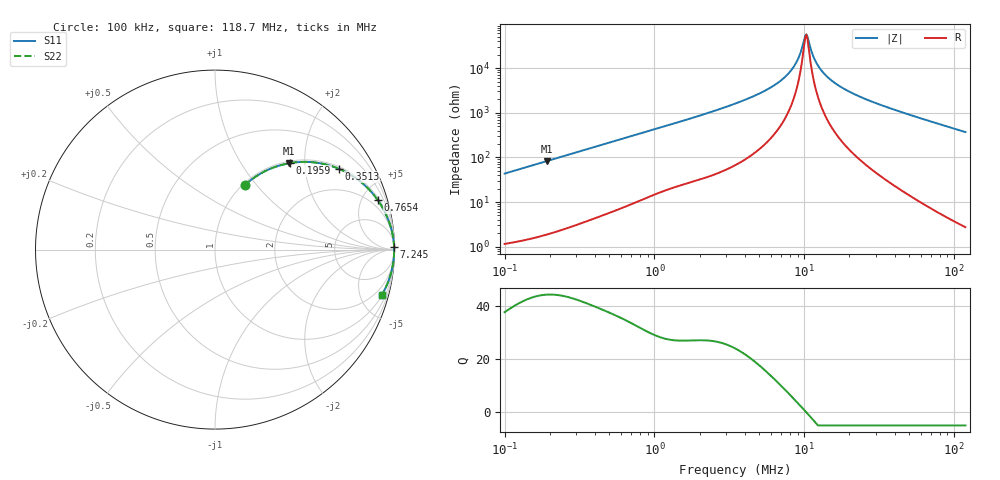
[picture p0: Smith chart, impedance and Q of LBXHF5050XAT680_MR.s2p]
! LBXHF5050XAT680_MR  S-PARAMETER MODEL  ( Standard Model )
! Model Generated by TAIYO YUDEN Corporation (http://www.ty-top.com)
! Version 1.0
! TAIYO YUDEN Control No. 20221109
! Copyright(c) 2022 TAIYO YUDEN CO.,LTD. All Rights Reserved.
! Product Description (link to TY-COMPAS)
! https://ds.yuden.co.jp/TYCOMPAS/or/detail?pn=LBXHF5050XAT680MMR&u=M
! Products Name : Inductors
! Characteristics :
!  Inductance : 68 [uH] , SRF(min) : 8.0 [MHz] , DC Resistance(max) : 0.576 [Ohm]
!  Rated Current : Saturation  750 [mA] , Temp Rise  470 [mA]
!  Case Size : 5.0 x 5.0 / 0.197 x 0.197 [mm/inch] , Thickness : 3.1 / 0.122 [mm/inch]
!  (Conditions: Temperature = 25 [degC] , DC Bias Current = 0 [A])
! External Node Assignments :
!  1  o---GGG---o  2
! GND o---------o GND
! Frequency Range : 0.1MHz  -  118.695536MHz  [ 402 STEP ]
# MHz S RI R 50
! Freq[MHz].  S11 Real  S11 Imag  S21 Real  S21 Imag  S12 Real  S12 Imag  S22 Real  S22 Imag
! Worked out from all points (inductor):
!   401 points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, 100 kHz to 118.7 MHz, reference 50 ohm
!   read as one part in series: L = 68.8 uH near 103.6 kHz
!   highest Q = 44.3 at 192.5 kHz (marker M1), where L = 68.7 uH
!   self-resonance near 10.14 MHz
!   S11 on the Smith chart (normalised r, x): 100 kHz: 1.02, +0.87; 195.9 kHz: 1.04, +1.69; 351.3 kHz: 1.07, +3.02; 765.4 kHz: 1.20, +6.53; 7.245 MHz: open; 118.7 MHz: 1.05, -7.39
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0.1  0.1646 0.3578  0.8354 -0.3578  0.8354 -0.3578  0.1646 0.3578
0.19248  0.4102 0.4807  0.5898 -0.4807  0.5898 -0.4807  0.4102 0.4807
0.195917  0.4185 0.4822  0.5815 -0.4822  0.5815 -0.4822  0.4185 0.4822
0.327316  0.6606 0.4617  0.3394 -0.4617  0.3394 -0.4617  0.6606 0.4617
0.351327  0.6905 0.4503  0.3095 -0.4503  0.3095 -0.4503  0.6905 0.4503
0.76542  0.9073 0.275  0.0927 -0.275  0.0927 -0.275  0.9073 0.275
1.07136  0.9476 0.206  0.0524 -0.206  0.0524 -0.206  0.9476 0.206
3.445222  0.9935 0.062  0.00645 -0.062  0.00645 -0.062  0.9935 0.062
5.362525  0.9969 0.0328  0.00312 -0.0328  0.00312 -0.0328  0.9969 0.0328
7.244907  0.9979 0.0169  0.00214 -0.0169  0.00214 -0.0169  0.9979 0.0169
8.056554  0.998 0.0116  0.00195 -0.0116  0.00195 -0.0116  0.998 0.0116
8.801967  0.9982 0.00738  0.00184 -0.00738  0.00184 -0.00738  0.9982 0.00738
9.281924  0.9982 0.00486  0.0018 -0.00486  0.0018 -0.00486  0.9982 0.00486
10.14071  0.9982 0.000685  0.00175 -0.000685  0.00175 -0.000685  0.9982 0.000685
10.50608  0.9983 -0.000983  0.00175 0.000983  0.00175 0.000983  0.9983 -0.000983
11.27678  0.9982 -0.00432  0.00175 0.00432  0.00175 0.00432  0.9982 -0.00432
12.10401  0.9982 -0.00769  0.00178 0.00769  0.00178 0.00769  0.9982 -0.00769
12.99193  0.9982 -0.0111  0.00184 0.0111  0.00184 0.0111  0.9982 -0.0111
16.06596  0.9978 -0.0217  0.00216 0.0217  0.00216 0.0217  0.9978 -0.0217
22.48756  0.9967 -0.0407  0.00333 0.0407  0.00333 0.0407  0.9967 -0.0407
36.91074  0.9923 -0.0775  0.00773 0.0775  0.00773 0.0775  0.9923 -0.0775
118.6955  0.9301 -0.2513  0.0699 0.2513  0.0699 0.2513  0.9301 -0.2513
